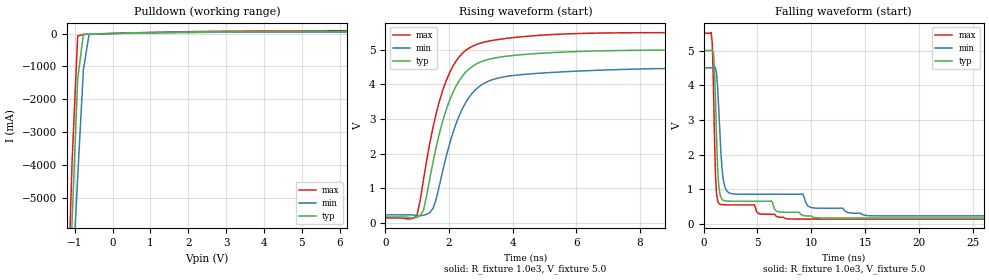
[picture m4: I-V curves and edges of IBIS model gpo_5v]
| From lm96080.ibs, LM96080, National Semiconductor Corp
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[Model] gpo_5v
Model_type Open_sink
Vmeas = 0.4V
Cref = 0.0pF
Rref = 1.0e3
Vref = 5.0V
C_comp   0.99pF   0.90pF   1.17pF
[Voltage Range]   5.0V   4.5V   5.5V
[Temperature Range]   25.0   125.0   -40.0
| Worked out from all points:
|   slope of the pulldown table from 0 to 0.75 V, typ, clamps not added: 38.1 ohm
|   rising waveform, R_fixture 1.0e3, V_fixture 5.0: 20-80 % time 906ps typ, 949ps min, 876ps max; typ from 0.17 V to 5 V
|   falling waveform, R_fixture 1.0e3, V_fixture 5.0: 20-80 % time 346ps typ, 611ps min, 261ps max; typ from 5 V to 0.17 V
[Pulldown]
-5V       -121.7A    -95.03A    -151.5A
-1.22V    -10.3A     -11.17A    -9.688A
-1.07V    -5.792A    -7.757A    -3.976A
-920mV    -1.386A    -4.392A    -75.54mA
-770mV    -30.71mA   -1.118A    -28.64mA
-620mV    -17.35mA   -31.1mA    -22.65mA
-305mV    -8.646mA   -5.705mA   -11.55mA
2.875V    53.3mA     36.61mA    67.81mA
10V       68.75mA    48.56mA    87.6mA
[Rising Waveform]
R_fixture=1.0e3
V_fixture=5.0
V_fixture_min=4.5
V_fixture_max=5.5
0s        170.3mV    231.6mV    140.1mV
1ns       162.2mV    211.2mV    244.4mV
1.2ns     376.8mV    219.9mV    1.258V
1.5ns     1.769V     419.9mV    2.771V
1.7ns     2.591V     1.089V     3.519V
2ns       3.497V     2.225V     4.301V
2.4ns     4.214V     3.258V     4.879V
3.2ns     4.712V     4.077V     5.241V
5.1ns     4.911V     4.338V     5.433V
99.95ns   5V         4.5V       5.5V
[Falling Waveform]
R_fixture=1.0e3
V_fixture=5.0
V_fixture_min=4.5
V_fixture_max=5.5
0s        5V         4.5V       5.5V
800ps     5.009V     4.5V       5.222V
1ns       4.49V      4.508V     2.601V
1.1ns     3.591V     4.509V     1.395V
1.4ns     1.12V      3.353V     598.8mV
1.7ns     714.3mV    1.617V     554.1mV
2.2ns     657.7mV    932.9mV    548.7mV
7.7ns     336.3mV    854mV      150.2mV
15.6ns    170.3mV    233.9mV    140.1mV
99.95ns   170.3mV    231.6mV    140.1mV
[Ramp]
R_load = 1.0e3
dV/dt_r   2.897827E0/9E-10   2.561003E0/1E-9   3.21593E0/9E-10
dV/dt_f   2.897832E0/3E-10   2.561008E0/6E-10   3.215933E0/3E-10
